[IBIS Ver]   3.2
[File Name]   sprm455.ibs
[File Rev]   1.0
[Date]   November 3, 2003
[Source]   File originated at Texas Instruments
[Copyright]   (c) 2003, Texas Instruments Inc.
[Component]   r2811pbk
[Manufacturer] Texas Instruments
[Package]
| Variable   Typ   Min   Max
R_pkg   0.063   0.061   0.064
L_pkg   2.512e-09   2.373e-10   2.8e-09
C_pkg   0.455e-13   0.4e-13   0.557e-13
[Pin] signal_name   model_name   R_pin   L_pin   C_pin
1   VDDAIO   NC   0.062 2.856e-09 0.429e-13
2   ADCINB0   NC   0.062 2.768e-09 0.518e-13
3   ADCINB1   NC   0.061 2.741e-09 0.555e-13
4   ADCINB2   NC   0.062 2.718e-09 0.542e-13
5   ADCINB3   NC   0.061 2.661e-09 0.499e-13
6   ADCINB4   NC   0.061 2.656e-09 0.526e-13
7   ADCINB5   NC   0.061 2.604e-09 0.498e-13
8   ADCINB6   NC   0.060 2.557e-09 0.432e-13
9   ADCINB7   NC   0.061 2.536e-09 0.437e-13
10   ADCREFM   NC   0.063 2.528e-09 0.411e-13
11   ADCREFP   NC   0.063 2.503e-09 0.376e-13
12   AVSSREFBG   NC   0.063 2.456e-09 0.366e-13
13   AVDDREFBG   NC   0.064 2.457e-09 0.374e-13
14   VDDA1   NC   0.065 2.457e-09 0.365e-13
15   VSSA1   NC   0.065 2.384e-09 0.330e-13
16   ADCRESEXT   NC   0.065 2.337e-09 0.356e-13
17   VSS   NC   0.065 2.341e-09 0.356e-13
18   MDRA   IDG09_OUO43_PS100  0.065 2.380e-09 0.329e-13
19   MDXA   IDG09_OUO43   0.065 2.466e-09 0.366e-13
20   VDD   NC   0.065 2.481e-09 0.376e-13
21   MCLKRA   IDG09_OUO43_PS100 0.064 2.479e-09 0.368e-13
22   MFSXA   IDG09_OUO43_PS100 0.063 2.500e-09 0.376e-13
23   MCLKXA   IDG09_OUO43_PS100 0.063 2.528e-09 0.412e-13
24   MFSRA   IDG09_OUO43_PS100 0.062 2.551e-09 0.439e-13
25   VDDIO   NC   0.062 2.591e-09 0.435e-13
26   VSS   NC   0.062 2.636e-09 0.502e-13
27   SPICLKA   IDG09_OUO43   0.062 2.663e-09 0.526e-13
28   SPISTEA   IDG09_OUO43   0.062 2.676e-09 0.500e-13
29   VDD   NC   0.062 2.731e-09 0.543e-13
30   VSS   NC   0.062 2.763e-09 0.557e-13
31   SPISIMOA   IDG09_OUO43   0.063 2.792e-09 0.520e-13
32   SPISOMIA   IDG09_OUO43   0.064 2.889e-09 0.432e-13
33   PWM7   IDG09_OUO43_PS100 0.062 2.856e-09 0.429e-13
34   PWM8   IDG09_OUO43_PS100 0.062 2.768e-09 0.518e-13
35   PWM9   IDG09_OUO43_PS100 0.061 2.741e-09 0.555e-13
36   PWM10   IDG09_OUO43_PS100  0.062 2.718e-09 0.542e-13
37   PWM11   IDG09_OUO43_PS100 0.061 2.661e-09 0.499e-13
38   PWM12   IDG09_OUO43_PS100 0.061 2.656e-09 0.526e-13
39   VSS   NC   0.061 2.604e-09 0.498e-13
40   T3PWM_T3CMP   IDG09_OUO43_PS100 0.060 2.557e-09 0.432e-13
41   T4PWM_T4CMP   IDG09_OUO43_PS100 0.061 2.536e-09 0.437e-13
42   VDD   NC   0.063 2.528e-09 0.411e-13
43   CAP4_QEP3   IDG09_OUO43_PS100 0.063 2.503e-09 0.376e-13
44   CAP5_QEP4   IDG09_OUO43_PS100 0.063 2.456e-09 0.366e-13
45   CAP6_QEPI2   IDG09_OUO43_PS100 0.064 2.457e-09 0.374e-13
46   C4TRIPn   IDG09_OUO43_PS100 0.065 2.457e-09 0.365e-13
47   C5TRIPn   IDG09_OUO43_PS100 0.065 2.384e-09 0.330e-13
48   C6TRIPn   IDG09_OUO43_PS100 0.065 2.337e-09 0.356e-13
49   VDDIO   NC   0.065 2.341e-09 0.356e-13
50   TEST2   NC   0.065 2.380e-09 0.329e-13
51   TEST1   NC   0.065 2.466e-09 0.366e-13
52   VDDIO   NC   0.065 2.481e-09 0.376e-13
53   VSS   NC   0.064 2.479e-09 0.368e-13
54   TDIRB   IDG09_OUO43_PS100 0.063 2.500e-09 0.376e-13
55   TCLKINB   IDG09_OUO43_PS100 0.063 2.528e-09 0.412e-13
56   VDD   NC   0.062 2.551e-09 0.439e-13
57   X2   NC   0.062 2.591e-09 0.435e-13
58   X1/XCLKIN   NC   0.062 2.636e-09 0.502e-13
59   VSS   NC   0.062 2.663e-09 0.526e-13
60   T3CTRIP_PDPINTBn IDG09_OUO43_PS100 0.062 2.676e-09 0.500e-13
61   T4CTRIPn/EVBSOCn IDG09_OUO43_PS100 0.062 2.731e-09 0.543e-13
62   VSS   NC   0.062 2.763e-09 0.557e-13
63   VDD   NC   0.063 2.792e-09 0.520e-13
64   CANTXA   IDG09_OUO43_PS100 0.064 2.889e-09 0.43205e-
65   CANRXA   IDG09_OUO43_PS100 0.062 2.856e-09 0.42905e-
66   SCITXDB   IDG09_OUO43   0.062 2.768e-09 0.518e-13
67   SCIRXDB   IDG09_OUO43   0.061 2.741e-09 0.555e-13
68   PWM1   IDG09_OUO43_PS100 0.062 2.718e-09 0.542e-13
69   PWM2   IDG09_OUO43_PS100 0.061 2.661e-09 0.499e-13
70   PWM3   IDG09_OUO43_PS100 0.061 2.656e-09 0.526e-13
71   PWM4   IDG09_OUO43_PS100 0.061 2.604e-09 0.498e-13
72   PWM5   IDG09_OUO43_PS100 0.060 2.557e-09 0.432e-13
73   VSS   NC   0.061 2.536e-09 0.437e-13
74   VDD   NC   0.063 2.528e-09 0.411e-13
75   PWM6   IDG09_OUO43_PS100 0.063 2.503e-09 0.376e-13
76   T1PWM_T1CMP   IDG09_OUO43_PS100 0.063 2.456e-09 0.366e-13
77   T2PWM_T2CMP   IDG09_OUO43_PS100 0.064 2.457e-09 0.374e-13
78   CAP1_QEP1   IDG09_OUO43_PS100 0.065 2.457e-09 0.365e-13
79   CAP2_QEP2   IDG09_OUO43_PS100 0.065 2.384e-09 0.330e-13
80   CAP3_QEPI1   IDG09_OUO43_PS100 0.065 2.337e-09 0.356e-13
81   T1CTRIP_PDPINTAn IDG09_OUO43_PS100 0.065 2.341e-09 0.356e-13
82   VDD   NC   0.065 2.380e-09 0.329e-13
83   VDDIO   NC   0.065 2.466e-09 0.366e-13
84   T2CTRIPn/EVASOCn IDG09_OUO43_PS100 0.065 2.481e-09 0.376e-13
85   TDIRA   IDG09_OUO43_PS100 0.064 2.479e-09 0.368e-13
86   TCLKINA   IDG09_OUO43_PS100 0.063 2.500e-09 0.376e-13
87   XCLKOUT   OUI83   00.063 2.528e-09 0.412e-13
88   VSS   NC   00.062 2.551e-09 0.439e-13
89   C1TRIPn   IDG09_OUO43_PS100 0.062 2.591e-09 0.435e-13
90   C2TRIPn   IDG09_OUO43_PS100 0.062 2.636e-09 0.502e-13
91   C3TRIPn   IDG09_OUO43_PS100 0.062 2.663e-09 0.526e-13
92   TMS   IDG09_PS100   00.062 2.676e-09 0.500e-13
93   TDO   OUI83   00.062 2.731e-09 0.543e-13
94   VDD   NC   00.062 2.763e-09 0.557e-13
95   VSS   NC   00.063 2.792e-09 0.520e-13
96   TDI   IDG09_PS100   00.064 2.889e-09 0.432e-13
97   TESTSEL   IDG09_PE100   00.062 2.856e-09 0.429e-13
98   TRSTn   IDG09_PE100   00.062 2.768e-09 0.518e-13
99   TCK   IDG09_PS100   00.061 2.741e-09 0.555e-13
100   EMU0   IDG09_OUI83_PS100 0.062 2.718e-09 0.542e-13
101   XF_XPLLDIS   IDG09_OUI83_PS100 0.061 2.661e-09 0.499e-13
102   VDD   NC   0.061 2.656e-09 0.526e-13
103   VSS   NC   0.061 2.604e-09 0.498e-13
104   VDDIO   NC   0.060 2.557e-09 0.432e-13
105   EMU1   IDG09_OUI83_PS100 0.061 2.536e-09 0.437e-132
106   XINT1_XBIOn   IDG09_OUO43   0.063 2.528e-09 0.411e-13
107   XNMI_XINT13   IDG09_OUO43_PS100 0.063 2.503e-09 0.376e-13
108   XINT2_ADCSOC   IDG09_OUO43   0.063 2.456e-09 0.366e-13
109   VSS   NC   0.064 2.457e-09 0.374e-13
110   VDD   NC   0.065 2.457e-09 0.365e-13
111   SCITXDA   IDG09_OUO43_PS100 0.065 2.384e-09 0.330e-13
112   SCIRXDA   IDG09_OUO43_PS100 0.065 2.337e-09 0.356e-13
113   XRSn   IDG09_OUM42_PS100 0.065 2.341e-09 0.356e-132
114   VDD1   NC   0.065 2.380e-09 0.329e-13
115   VSS1   NC   0.065 2.466e-09 0.366e-13
116   ADCBGREFIN   NC   0.065 2.481e-09 0.376e-13
117   VSSA2   NC   0.064 2.479e-09 0.368e-13
118   VDDA2   NC   0.063 2.500e-09 0.376e-13
119   ADCINA7   NC   0.063 2.528e-09 0.412e-13
120   ADCINA6   NC   0.062 2.551e-09 0.439e-13
121   ADCINA5   NC   0.062 2.591e-09 0.435e-13
122   ADCINA4   NC   0.062 2.636e-09 0.502e-13
123   ADCINA3   NC   0.062 2.663e-09 0.526e-13
124   ADCINA2   NC   0.062 2.676e-09 0.500e-13
125   ADCINA1   NC   0.062 2.731e-09 0.543e-13
126   ADCINA0   NC   0.062 2.763e-09 0.557e-13
127   ADCLO   NC   0.063 2.792e-09 0.520e-13
128   VSSAIO   NC   0.064 2.889e-09 0.432e-13
| End of package information
|   GS30 Cell IDG09_PE100
|   Component IDG09_PE100
[Component]   IDG09_PE100
[Manufacturer]   Texas Instruments
[Package]
|  variable   typ   min   max
R_pkg   0   0   0
L_pkg   0   0   0
C_pkg   0   0   0
[Pin]   signal_name   model_name   R_pin   L_pin   C_pin
VDDS   VDDS   POWER
VSS   VSS   GND
PAD   PAD   IDG09_PE100
[Model Selector] IDG09_PE100
9_PE100_PULLDOWN_2P5  Cell operated at 2.5(nom)
|IDG09_PE100_PULLDOWN_2P5; BUFFER WITH WEAK_PULLDOWN_ON
PE100_NOPULLDOWN_2P5  Cell operated at 2.5(nom)
|IDG09_PE100_NOPULLDOWN_2P5; BUFFER OPERATING IN NORMMAL MODE WITHOUT PULLD
|OWN
9_PE100_PULLDOWN_3P3  Cell operated at 3.3(nom)
|IDG09_PE100_PULLDOWN_3P3; BUFFER WITH WEAK_PULLDOWN_ON
PE100_NOPULLDOWN_3P3  Cell operated at 3.3(nom)
|IDG09_PE100_NOPULLDOWN_3P3; BUFFER OPERATING IN NORMMAL MODE WITHOUT PULLD
|OWN
_PE100_PULLDOWN_2P75  Cell operated at 2.75(nom)
|IDG09_PE100_PULLDOWN_2P75; BUFFER WITH WEAK_PULLDOWN_ON
E100_NOPULLDOWN_2P75  Cell operated at 2.75(nom)
[Component]   IDG09_OUO43
[Manufacturer]   Texas Instruments
[Package]
|  variable   typ   min   max
R_pkg   0   0   0
L_pkg   0   0   0
C_pkg   0   0   0
[Pin]   signal_name   model_name   R_pin   L_pin   C_pin
VSS   VSS   GND
VDDS   VDDS   POWER
PAD   PAD   IDG09_OUO43
[Model Selector] IDG09_OUO43
IDG09_OUO43_2P5  Cell operated at 2.5(nom)
|IDG09_OUO43_2P5; DEFAULT
IDG09_OUO43_3P3  Cell operated at 3.3(nom)
|IDG09_OUO43_3P3; DEFAULT
IDG09_OUO43_2P75  Cell operated at 2.75(nom)
|   Component IDG09_PS100
[Component]   IDG09_PS100
[Manufacturer]   Texas Instruments
[Package]
|  variable   typ   min   max
R_pkg   0   0   0
L_pkg   0   0   0
C_pkg   0   0   0
[Pin]   signal_name   model_name   R_pin   L_pin   C_pin
VDDS   VDDS   POWER
VSS   VSS   GND
PAD   PAD   IDG09_PS100
[Model Selector] IDG09_PS100
G09_PS100_PULLUP_2P5  Cell operated at 2.5(nom)
|IDG09_PS100_PULLUP_2P5; BUFFER WITH WEAK_PULLUP_ON
9_PS100_NOPULLUP_2P5  Cell operated at 2.5(nom)
|IDG09_PS100_NOPULLUP_2P5; BUFFER OPERATING IN NORMMAL MODE WITHOUT PULLUP
G09_PS100_PULLUP_3P3  Cell operated at 3.3(nom)
|IDG09_PS100_PULLUP_3P3; BUFFER WITH WEAK_PULLUP_ON
9_PS100_NOPULLUP_3P3  Cell operated at 3.3(nom)
|IDG09_PS100_NOPULLUP_3P3; BUFFER OPERATING IN NORMMAL MODE WITHOUT PULLUP
09_PS100_PULLUP_2P75  Cell operated at 2.75(nom)
|IDG09_PS100_PULLUP_2P75; BUFFER WITH WEAK_PULLUP_ON
_PS100_NOPULLUP_2P75  Cell operated at 2.75(nom)
|   Component OUI83
[Component]   OUI83
[Manufacturer]   Texas Instruments
[Package]
|  variable   typ   min   max
R_pkg   0   0   0
L_pkg   0   0   0
C_pkg   0   0   0
[Pin]   signal_name   model_name   R_pin   L_pin   C_pin
VSS   VSS   GND
VDDS   VDDS   POWER
Y   Y   OUI83
[Model Selector] OUI83
OUI83_2P5  Cell operated at 2.5(nom)
|OUI83_2P5; DEFAULT
OUI83_3P3  Cell operated at 3.3(nom)
|OUI83_3P3; DEFAULT
OUI83_2P75  Cell operated at 2.75(nom)
|   Component IDG09_OUI83_PS100
[Component]   IDG09_OUI83_PS100
[Manufacturer]   Texas Instruments
[Package]
|  variable   typ   min   max
R_pkg   0   0   0
L_pkg   0   0   0
C_pkg   0   0   0
[Pin]   signal_name   model_name   R_pin   L_pin   C_pin
VSS   VSS   GND
VDDS   VDDS   POWER
PAD   PAD   IDG09_OUI83_PS100
[Model Selector] IDG09_OUI83_PS100
UI83_PS100_PU_ON_2P5  Cell operated at 2.5(nom)
|IDG09_OUI83_PS100_PU_ON_2P5; BUFFER WITH WEAK_PULLUP_ON
I83_PS100_PU_OFF_2P5  Cell operated at 2.5(nom)
|IDG09_OUI83_PS100_PU_OFF_2P5; BUFFER IN NORMAL MODE WITH PULLUP AND PUL
|LDOWN OFF
UI83_PS100_PU_ON_3P3  Cell operated at 3.3(nom)
|IDG09_OUI83_PS100_PU_ON_3P3; BUFFER WITH WEAK_PULLUP_ON
I83_PS100_PU_OFF_3P3  Cell operated at 3.3(nom)
|IDG09_OUI83_PS100_PU_OFF_3P3; BUFFER IN NORMAL MODE WITH PULLUP AND PUL
|LDOWN OFF
I83_PS100_PU_ON_2P75  Cell operated at 2.75(nom)
|IDG09_OUI83_PS100_PU_ON_2P75; BUFFER WITH WEAK_PULLUP_ON
83_PS100_PU_OFF_2P75  Cell operated at 2.75(nom)
|   Component IDG09_OUO43_PS100
[Component]   IDG09_OUO43_PS100
[Manufacturer]   Texas Instruments
[Package]
|  variable   typ   min   max
R_pkg   0   0   0
L_pkg   0   0   0
C_pkg   0   0   0
[Pin]   signal_name   model_name   R_pin   L_pin   C_pin
VSS   VSS   GND
VDDS   VDDS   POWER
PAD   PAD   IDG09_OUO43_PS100
[Model Selector] IDG09_OUO43_PS100
UO43_PS100_PU_ON_2P5  Cell operated at 2.5(nom)
|IDG09_OUO43_PS100_PU_ON_2P5; BUFFER WITH WEAK_PULLUP_ON
O43_PS100_PU_OFF_2P5  Cell operated at 2.5(nom)
|IDG09_OUO43O43_PS100_PU_OFF_2P5; BUFFER IN NORMAL MODE WITH PULLUP
| OFF
UO43_PS100_PU_ON_3P3  Cell operated at 3.3(nom)
|IDG09_OUO43_PS100_PU_ON_3P3; BUFFER WITH WEAK_PULLUP_ON
O43_PS100_PU_OFF_3P3  Cell operated at 3.3(nom)
|IDG09_OUO43_PS100_PU_OFF_3P3; BUFFER IN NORMAL MODE WITH PULLUP
| OFF
O43_PS100_PU_ON_2P75  Cell operated at 2.75(nom)
|IDG09_OUO43_PS100_PU_ON_2P75; BUFFER WITH WEAK_PULLUP_ON
43_PS100_PU_OFF_2P75  Cell operated at 2.75(nom)
|   Component IDG09_OUM42_PS100
[Component]   IDG09_OUM42_PS100
[Manufacturer]   Texas Instruments
[Package]
|  variable   typ   min   max
R_pkg   0   0   0
L_pkg   0   0   0
C_pkg   0   0   0
[Pin]   signal_name   model_name   R_pin   L_pin   C_pin
VSS   VSS   GND
VDDS   VDDS   POWER
PAD   PAD   IDG09_OUM42_PS100
[Model Selector] IDG09_OUM42_PS100
UM42_PS100_PU_ON_2P5  Cell operated at 2.5(nom)
|IDG09_OUM42_PS100_PU_ON_2P5; BUFFER WITH WEAK_PULLUP_ON
M42_PS100_PU_OFF_2P5  Cell operated at 2.5(nom)
|IDG09_OUM42_PS100_PU_OFF_2P5; BUFFER IN NORMAL MODE WITH PULLUP OFF
UM42_PS100_PU_ON_3P3  Cell operated at 3.3(nom)
|IDG09_OUM42_PS100_PU_ON_3P3; BUFFER WITH WEAK_PULLUP_ON
M42_PS100_PU_OFF_3P3  Cell operated at 3.3(nom)
|IDG09_OUM42_PS100_PU_OFF_3P3; BUFFER IN NORMAL MODE WITH PULLUP OFF
M42_PS100_PU_ON_2P75  Cell operated at 2.75(nom)
|IDG09_OUM42_PS100_PU_ON_2P75; BUFFER WITH WEAK_PULLUP_ON
42_PS100_PU_OFF_2P75  Cell operated at 2.75(nom)
| Models and submodels in the file (36): 9_PE100_PULLDOWN_2P5 (Input), PE100_NOPULLDOWN_2P5 (Input), 9_PE100_PULLDOWN_3P3 (Input), PE100_NOPULLDOWN_3P3 (Input), _PE100_PULLDOWN_2P75 (Input), E100_NOPULLDOWN_2P75 (Input), IDG09_OUO43_2P5 (I/O), IDG09_OUO43_3P3 (I/O), IDG09_OUO43_2P75 (I/O), G09_PS100_PULLUP_2P5 (Input), 9_PS100_NOPULLUP_2P5 (Input), G09_PS100_PULLUP_3P3 (Input), 9_PS100_NOPULLUP_3P3 (Input), 09_PS100_PULLUP_2P75 (Input), _PS100_NOPULLUP_2P75 (Input), OUI83_2P5 (3-state), OUI83_3P3 (3-state), OUI83_2P75 (3-state), UI83_PS100_PU_ON_2P5 (I/O), I83_PS100_PU_OFF_2P5 (I/O), UI83_PS100_PU_ON_3P3 (I/O), I83_PS100_PU_OFF_3P3 (I/O), I83_PS100_PU_ON_2P75 (I/O), 83_PS100_PU_OFF_2P75 (I/O), UO43_PS100_PU_ON_2P5 (I/O), O43_PS100_PU_OFF_2P5 (I/O), UO43_PS100_PU_ON_3P3 (I/O), O43_PS100_PU_OFF_3P3 (I/O), O43_PS100_PU_ON_2P75 (I/O), 43_PS100_PU_OFF_2P75 (I/O), UM42_PS100_PU_ON_2P5 (I/O_open_drain), M42_PS100_PU_OFF_2P5 (I/O_open_drain), UM42_PS100_PU_ON_3P3 (I/O_open_drain), M42_PS100_PU_OFF_3P3 (I/O_open_drain), M42_PS100_PU_ON_2P75 (I/O_open_drain), 42_PS100_PU_OFF_2P75 (I/O_open_drain)
